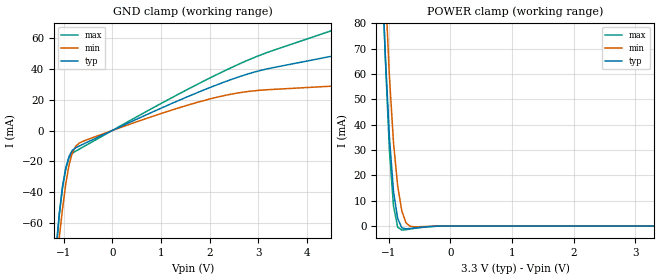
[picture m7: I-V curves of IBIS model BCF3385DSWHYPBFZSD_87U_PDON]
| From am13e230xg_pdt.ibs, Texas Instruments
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|   Model BCF3385DSWHYPBFZSD_87U_PDON
[Model] BCF3385DSWHYPBFZSD_87U_PDON
Model_type Input
Polarity   Non-Inverting
Enable   Active-High
Vinl =  0.990V
Vinh =  2.310V
C_comp   0.593pF   0.545pF   0.644pF
[Model Spec]
Vinh   2.310V   2.079V   2.541V
Vinl   0.990V   0.891V   1.089V
[Temperature Range]   25.000   0.155k   -40.000
[Voltage Range]   3.300V   2.970V   3.630V
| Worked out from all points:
|   GND clamp passes 1 mA (typ) near -0.07 V on its own axis
|   POWER clamp passes 1 mA (typ) near -0.67 V on its own axis
[GND_clamp]
|Voltage   I(typ)   I(min)   I(max)
-3.3V     -1.01A     -884.3mA   -1.279A
-1.156V   -76.89mA   -90.36mA   -80.6mA
-1.089V   -54.37mA   -69.72mA   -54.78mA
-1.022V   -36.28mA   -50.84mA   -37.14mA
-955mV    -24.21mA   -34.64mA   -25.19mA
-888mV    -16.78mA   -22.39mA   -17.6mA
-821mV    -12.89mA   -14.57mA   -14.77mA
-754mV    -11.24mA   -10.36mA   -13.42mA
1.189V    17.03mA    12.89mA    20.65mA
2.328V    31.69mA    22.8mA     38.95mA
3.266V    40.46mA    26.55mA    51.42mA
6.6V      60.98mA    32.35mA    86.97mA
[POWER_clamp]
|Voltage   I(typ)   I(min)   I(max)
-3.3V     1.723A     1.974A     1.841A
-1.122V   107.5mA    137.4mA    111mA
-1.055V   67.99mA    94.99mA    66.85mA
-988mV    35.14mA    59.2mA     30.08mA
-921mV    13.56mA    32.75mA    7.897mA
-854mV    2.974mA    15.88mA    -390.6uA
-787mV    -679.9uA   5.996mA    -1.606mA
-720mV    -1.105mA   1.301mA    -1.421mA
-653mV    -960.1uA   -90.68uA   -1.168mA
-586mV    -772.1uA   -323.6uA   -929.5uA
-117mV    0A         0A         0A
3.3V      0A         0A         0A
